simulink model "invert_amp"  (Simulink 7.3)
settings: Solver=ode45  StartTime=0.0  StopTime=0.002  MaxStep=0.00002  RelTol=1e-3
libraries: fl_lib x8, nesl_utility x3

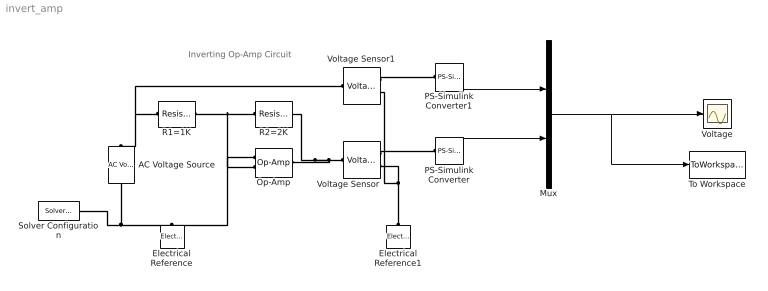
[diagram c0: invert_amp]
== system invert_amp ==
  note: Inverting Op-Amp Circuit
  AC Voltage Source : fl_lib/Electrical/Electrical Sources/AC Voltage Source  DialogController=NetworkEngine.DynNeDlgSource  SystemSampleTime=-1  amp=0.1 V  shift=0 rad  omega=2*pi*1000 rad/s  i_Log=off  v_Log=off  LocalVarNames=|current|voltage|power  LocalVarDescs=|Current (A)|Voltage (V)|Power (W)  LocalVarLogging=[0 0 0]
  Electrical Reference : fl_lib/Electrical/Electrical Elements/Electrical Reference  DialogController=NetworkEngine.DynNeDlgSource  SystemSampleTime=-1  i_Log=off  LocalVarNames=|i  LocalVarDescs=|i  LocalVarLogging=[]
  Electrical Reference1 : fl_lib/Electrical/Electrical Elements/Electrical Reference  DialogController=NetworkEngine.DynNeDlgSource  SystemSampleTime=-1  i_Log=off  LocalVarNames=|i  LocalVarDescs=|i  LocalVarLogging=[]
  Mux : Mux  Inputs=2
  Op-Amp : fl_lib/Electrical/Electrical Elements/Op-Amp  DialogController=NetworkEngine.DynNeDlgSource  SystemSampleTime=-1  i1_Log=off  v1_Log=off  outI_Log=off  LocalVarNames=|i1|v1|outI  LocalVarDescs=|i1|v1|outI  LocalVarLogging=[]
  PS-Simulink Converter : nesl_utility/PS-Simulink Converter  DialogController=NetworkEngine.DynNeUtilDlgSource  SystemSampleTime=-1  PhysicalDomain=network_engine_domain  LeftPortType=input  RightPortType=output  SubClassName=ps_output  Unit=1  AffineConversion=off
  PS-Simulink Converter1 : nesl_utility/PS-Simulink Converter  DialogController=NetworkEngine.DynNeUtilDlgSource  SystemSampleTime=-1  PhysicalDomain=network_engine_domain  LeftPortType=input  RightPortType=output  SubClassName=ps_output  Unit=1  AffineConversion=off
  R1=1K : fl_lib/Electrical/Electrical Elements/Resistor  DialogController=NetworkEngine.DynNeDlgSource  SystemSampleTime=-1  R=1e3 Ohm  i_Log=off  v_Log=off  LocalVarNames=|current|voltage|power  LocalVarDescs=|Resistor current (A)|Voltage across resistor (V)|Power (W)  LocalVarLogging=[0 0 0]
  R2=2K : fl_lib/Electrical/Electrical Elements/Resistor  DialogController=NetworkEngine.DynNeDlgSource  SystemSampleTime=-1  R=2e3 Ohm  i_Log=off  v_Log=off  LocalVarNames=|current|voltage|power  LocalVarDescs=|Resistor current (A)|Voltage across resistor (V)|Power (W)  LocalVarLogging=[0 0 0]
  Solver Configuration : nesl_utility/Solver Configuration  DialogController=NetworkEngine.DynNeUtilDlgSource  SystemSampleTime=-1  PhysicalDomain=network_engine_domain  LeftPortType=input  RightPortType=generic  SubClassName=solver  Accelerate=off  Profile=off  ResidualTolerance=1e-9  MaxNonlinIter=12  MaxModeIter=2  DoFixedCost=off  DoDC=off  LinearAlgebra=Sparse
  To Workspace : ToWorkspace  VariableName=sorties  SampleTime=-1  SaveFormat=Array
  Voltage : Scope
  Voltage Sensor : fl_lib/Electrical/Electrical Sensors/Voltage Sensor  DialogController=NetworkEngine.DynNeDlgSource  SystemSampleTime=-1  i1_Log=off  v1_Log=off  LocalVarNames=|i1|v1  LocalVarDescs=|i1|v1  LocalVarLogging=[]
  Voltage Sensor1 : fl_lib/Electrical/Electrical Sensors/Voltage Sensor  DialogController=NetworkEngine.DynNeDlgSource  SystemSampleTime=-1  i1_Log=off  v1_Log=off  LocalVarNames=|i1|v1  LocalVarDescs=|i1|v1  LocalVarLogging=[]
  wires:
  PS-Simulink Converter/1 -> Mux/2
  PS-Simulink Converter1/1 -> Mux/1
  Mux/1 -> Voltage/1, To Workspace/1
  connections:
  Electrical Reference/LConn1 -- AC Voltage Source/RConn1 -- Solver Configuration/RConn1 -- Op-Amp/LConn1
  R1=1K/LConn1 -- AC Voltage Source/LConn1 -- Voltage Sensor1/LConn1
  Op-Amp/LConn2 -- R1=1K/RConn1 -- R2=2K/LConn1
  Voltage Sensor/LConn1 -- R2=2K/RConn1 -- Op-Amp/RConn1
  Electrical Reference1/LConn1 -- Voltage Sensor/RConn2 -- Voltage Sensor1/RConn2
  Voltage Sensor/RConn1 -- PS-Simulink Converter/LConn1
  Voltage Sensor1/RConn1 -- PS-Simulink Converter1/LConn1
